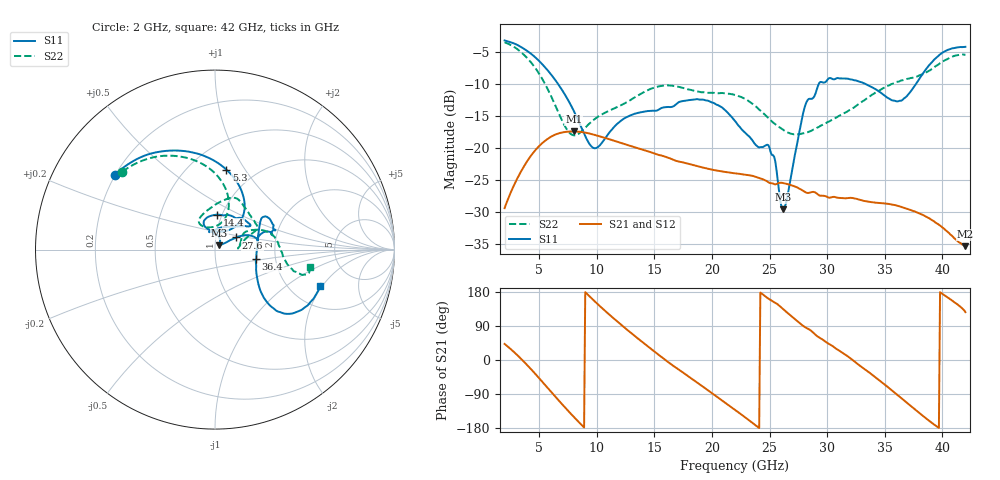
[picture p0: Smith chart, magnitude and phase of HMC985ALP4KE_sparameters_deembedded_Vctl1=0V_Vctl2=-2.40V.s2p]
!s2p File: Measurements: S11, S21, S12, S22
# GHz S dB R 50.0
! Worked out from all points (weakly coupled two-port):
!   401 points, 2 GHz to 42 GHz, reference 50 ohm
!   highest |S21| = -17.39 dB at 8 GHz (marker M1); lowest = -35.4 dB at 42 GHz (marker M2)
!   lowest |S11| = -29.6 dB at 26.2 GHz (marker M3), VSWR 1.07, Z = 52.3 + j2.49 ohm
!   |S11| at or under -10 dB: 6.654 GHz to 29.26 GHz (22.61 GHz wide, 126 % of centre); 33.37 GHz to 37.7 GHz (4.323 GHz wide, 12.2 % of centre)
!   |S22| runs from -18.0 to -3.4 dB; largest |S21 - S12| = 0.00057
!   S11 on the Smith chart (normalised r, x): 2 GHz: 0.20, +0.32; 5.3 GHz: 0.74, +0.83; 14.4 GHz: 0.95, +0.38; 27.6 GHz: 1.25, +0.17; 36.4 GHz: 1.58, -0.18; 42 GHz: 2.91, -1.91
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2  -3.14 143.1  -29.40 42.4  -29.39 42.4  -3.42 139.9
3.5  -4.25 116.2  -23.43 1.0  -23.44 0.9  -5.09 111.0
5.3  -6.93 81.9  -19.17 -58.4  -19.20 -58.5  -9.27 80.1
8  -14.16 48.1  -17.39 -150.0  -17.38 -149.9  -18.00 96.9
8.7  -16.94 52.4  -17.49 -171.8  -17.50 -171.9  -17.34 112.9
9.9  -20.02 87.2  -17.98 152.6  -17.97 152.6  -15.35 120.8
12.2  -15.58 112.2  -19.26 90.8  -19.24 90.9  -13.21 103.1
14.4  -14.21 87.0  -20.48 36.5  -20.46 36.6  -10.96 78.8
15.4  -13.95 73.4  -21.09 13.1  -21.10 13.0  -10.33 71.6
19.3  -12.44 34.1  -23.09 -72.2  -23.11 -72.2  -11.26 42.9
22  -15.76 52.3  -23.95 -131.4  -23.98 -131.4  -11.68 26.2
25  -19.98 98.8  -25.46 160.0  -25.43 160.1  -15.49 17.3
26.2  -29.58 45.8  -25.49 133.7  -25.53 133.6  -17.18 8.0
27.6  -17.35 29.8  -26.38 97.5  -26.38 97.5  -17.78 3.3
28.1  -13.29 20.9  -26.90 86.3  -26.93 86.4  -17.63 5.0
28.7  -12.26 13.0  -26.88 74.7  -26.88 74.7  -17.20 9.2
31  -9.05 23.3  -27.80 25.6  -27.79 25.5  -14.99 28.7
33.3  -9.94 34.2  -28.31 -25.1  -28.30 -25.2  -12.43 27.2
35.4  -12.27 12.0  -28.77 -74.7  -28.75 -74.7  -10.16 18.3
36.4  -12.58 -13.2  -29.19 -99.7  -29.23 -99.8  -9.42 12.5
39.5  -5.81 -43.4  -31.77 -174.9  -31.74 -175.1  -7.08 -14.1
42  -4.14 -19.0  -35.37 126.3  -35.35 126.3  -5.35 -10.3
